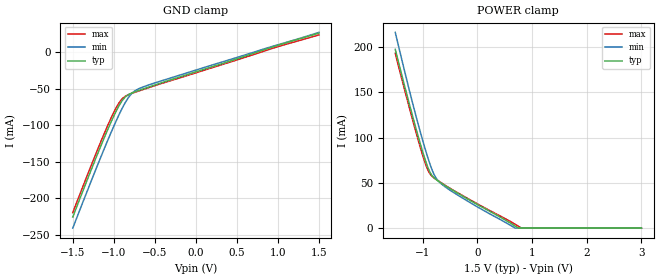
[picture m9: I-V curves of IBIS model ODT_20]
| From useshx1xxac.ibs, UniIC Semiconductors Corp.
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|   Model ODT_20
[Model]  ODT_20
Model_type   Input
Polarity   Non-Inverting
Vinl =   0.600000V
Vinh =   0.900000V
C_comp   1.3900pF   1.3640pF   1.5600pF
[Temperature Range]   25.0000   95.0000   0.0
[Voltage Range]   1.5000V   1.4000V   1.6000V
[GND_clamp]
|Voltage   I(typ)   I(min)   I(max)
-1.5V     -225.7mA   -240.8mA   -219.7mA
-1.18V    -134.4mA   -149.7mA   -128.5mA
-1.06V    -102.3mA   -117mA     -96.79mA
-980mV    -82.64mA   -96.28mA   -77.86mA
-940mV    -73.96mA   -86.48mA   -69.95mA
-900mV    -66.63mA   -77.27mA   -63.96mA
-860mV    -61.28mA   -68.92mA   -60.29mA
-780mV    -55.87mA   -56.37mA   -56.42mA
-740mV    -54.15mA   -52.67mA   -54.86mA
-460mV    -43.35mA   -40.68mA   -44.38mA
980mV     8.643mA    9.484mA    6.84mA
1.5V      26.1mA     27.08mA    23.55mA
[POWER_clamp]
|Voltage   I(typ)   I(min)   I(max)
-1.5V     197.5mA    216.3mA    193.4mA
-1.18V    123.1mA    137.5mA    119mA
-1.04V    92.71mA    105.8mA    88.7mA
-940mV    73.14mA    84.82mA    69.67mA
-860mV    61.13mA    69.79mA    59.52mA
-780mV    55.02mA    58.04mA    55.01mA
-720mV    52.28mA    52.59mA    52.52mA
-640mV    49mA       48.07mA    49.36mA
0V        26.1mA     23.52mA    26.86mA
600mV     5.719mA    3.337mA    7.53mA
752.6mV   0A         NA         NA
3V        0A         0A         0A
